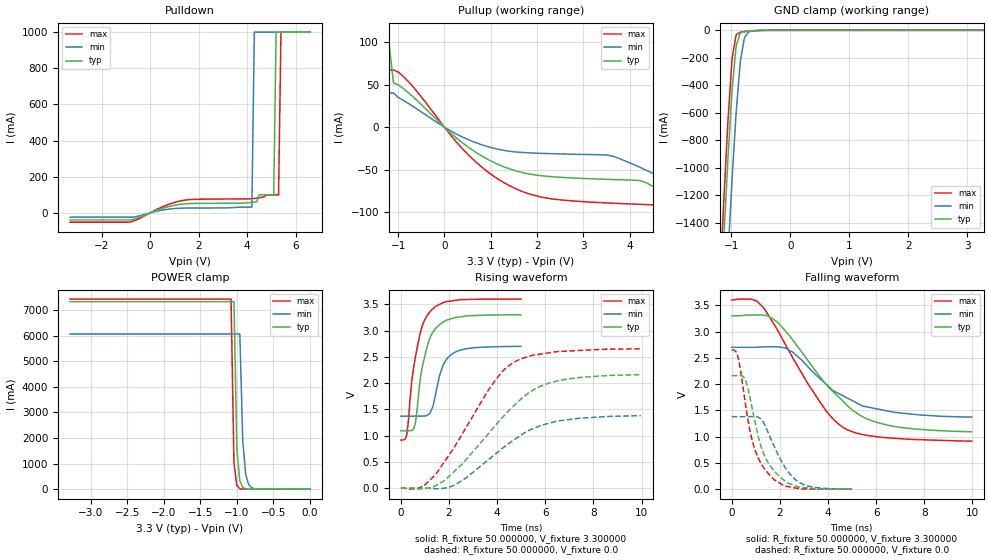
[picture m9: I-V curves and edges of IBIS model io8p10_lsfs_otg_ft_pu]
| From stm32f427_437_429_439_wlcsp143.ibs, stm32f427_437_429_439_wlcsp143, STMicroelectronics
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|   Model io8p10_lsfs_otg_ft_pu
[Model]  io8p10_lsfs_otg_ft_pu
Model_type I/O
Polarity   Non-Inverting
Enable   Active-Low
Vinl =   0.990000V
Vinh =   2.310000V
Vmeas =  1.650000V
Cref =   40.000000pF
Rref =   100.000000M
Vref =   0.0V
C_comp   8.196500pF   7.968500pF   8.492600pF
[Temperature Range]   25.000000   0.125000k   -40.000000
[Pullup Reference]   3.300000V   2.700000V   3.600000V
[Pulldown Reference]   0.0V   0.0V   0.0V
[POWER Clamp Reference]   3.300000V   2.700000V   3.600000V
[GND Clamp Reference]   0.0V   0.0V   0.0V
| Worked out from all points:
|   slope of the pulldown table from 0 to 0.495 V, typ, clamps not added: 20.1 ohm
|   slope of the pullup table from 0 to 0.495 V, typ, clamps not added: 21.8 ohm
|   GND clamp passes 1 mA (typ) near -0.52 V on its own axis
|   POWER clamp passes 1 mA (typ) near -0.80 V on its own axis
|   rising waveform, R_fixture 50.000000, V_fixture 3.300000: 20-80 % time 526ps typ, 499ps min, 529ps max; typ from 1.09 V to 3.3 V
|   rising waveform, R_fixture 50.000000, V_fixture 0.0: 20-80 % time 2.59ns typ, 2.41ns min, 2.19ns max; typ from 0.001 V to 2.16 V
|   falling waveform, R_fixture 50.000000, V_fixture 3.300000: 20-80 % time 2.44ns typ, 2.26ns min, 2.13ns max; typ from 3.3 V to 1.09 V
|   falling waveform, R_fixture 50.000000, V_fixture 0.0: 20-80 % time 849ps typ, 952ps min, 758ps max; typ from 2.16 V to 0.001 V
[Pulldown]
|Voltage   I(typ)   I(min)   I(max)
-3.3V     -38.65mA   -23.43mA   -51.3mA
-900mV    -38.65mA   -23.43mA   -51.3mA
1.4V      49.88mA    26.66mA    69.84mA
4.2V      58.43mA    32mA       78.86mA
4.3V      60.2mA     1A         80.13mA
4.4V      62mA       1A         81.72mA
4.5V      100mA      1A         83.79mA
5.1V      100mA      1A         100mA
5.2V      1A         1A         100mA
5.3V      1A         1A         100mA
5.4V      1A         1A         1A
6.6V      1A         1A         1A
[Pullup]
|Voltage   I(typ)   I(min)   I(max)
-3.3V     100mA      1A         67mA
-1.6V     100mA      1A         67mA
-1.5V     100mA      40mA       67mA
-1.2V     100mA      40mA       67mA
-1.1V     52mA       40mA       67mA
800mV     -33.66mA   -20.62mA   -46.63mA
2V        -56.45mA   -30.57mA   -80.98mA
3.5V      -61.24mA   -32.7mA    -88.93mA
4.2V      -62.55mA   -46.6mA    -90.52mA
4.9V      -82mA      -66mA      -102.3mA
5.5V      -103mA     -66mA      -126.2mA
6.6V      -103mA     -66mA      -139mA
[GND_clamp]
|Voltage   I(typ)   I(min)   I(max)
-3.3V     -9.479A    -9.465A    -9.974A
-1.2V     -2.125A    -2.854A    -1.857A
-1.13V    -1.511A    -2.236A    -1.236A
-1.06V    -933.3mA   -1.641A    -660.9mA
-990mV    -433.3mA   -1.082A    -206.9mA
-920mV    -110.3mA   -591mA     -31.45mA
-850mV    -19.78mA   -226.7mA   -13.65mA
-780mV    -8.311mA   -53.93mA   -9.506mA
-710mV    -5.285mA   -11.94mA   -6.262mA
-640mV    -3.232mA   -4.282mA   -3.577mA
3.28V     0A         0A         0A
[POWER_clamp]
|Voltage   I(typ)   I(min)   I(max)
-3.28V    7.329A     6.064A     7.43A
-1.08V    7.329A     6.064A     7.43A
-1.04V    7.329A     6.064A     1.015A
-1V       1.545A     6.064A     138.8mA
-960mV    325.8mA    6.064A     19.13mA
-920mV    68.77mA    1.89A      2.772mA
-880mV    14.59mA    589.1mA    520.3uA
-840mV    3.154mA    183.6mA    196.4uA
-800mV    734.4uA    57.27mA    136.6uA
-720mV    96.98uA    5.605mA    116.7uA
0V        0A         0A         0A
[Ramp]
| variable   typ   min   max
dV/dt_r  1.28451/2.59000n   0.82114/2.39692n   1.58763/2.18976n
dV/dt_f  1.29996/2.41613n   0.78216/2.23662n   1.59709/2.12461n
R_load = 50.000000
[Rising Waveform]
R_fixture= 50.000000
V_fixture= 3.300000
V_fixture_min= 2.700000
V_fixture_max= 3.600000
|time   V(typ)   V(min)   V(max)
0s        1.092V     1.372V     915.8mV
250.2ps   1.092V     1.372V     1.026V
460.5ps   1.1V       1.372V     2.071V
540.5ps   1.14V      1.372V     2.323V
610.6ps   1.262V     1.372V     2.511V
890.9ps   2.306V     1.372V     3.093V
1.251ns   2.902V     1.474V     3.38V
1.752ns   3.161V     2.343V     3.53V
2.142ns   3.234V     2.56V      3.567V
4.985ns   3.3V       2.7V       3.6V
[Rising Waveform]
R_fixture= 50.000000
V_fixture= 0.0
V_fixture_min= 0.0
V_fixture_max= 0.0
|time   V(typ)   V(min)   V(max)
0s        1.084mV    1.041mV    1.065mV
760.8ps   -15.37mV   1.053mV    5.82mV
1.441ns   47.59mV    -11.43mV   259.2mV
2.242ns   330mV      61.26mV    795.7mV
3.704ns   1.074V     566.8mV    1.913V
4.224ns   1.349V     760.4mV    2.224V
4.705ns   1.574V     921.8mV    2.4V
5.526ns   1.877V     1.14V      2.534V
6.466ns   2.038V     1.276V     2.599V
9.97ns    2.161V     1.38V      2.653V
[Falling Waveform]
R_fixture= 50.000000
V_fixture= 3.300000
V_fixture_min= 2.700000
V_fixture_max= 3.600000
|time   V(typ)   V(min)   V(max)
0s        3.3V       2.7V       3.6V
840.8ps   3.315V     2.7V       3.614V
1.341ns   3.308V     2.709V     3.444V
1.962ns   3.15V      2.706V     2.977V
2.543ns   2.833V     2.605V     2.495V
3.904ns   2.007V     2.004V     1.502V
4.625ns   1.673V     1.777V     1.177V
5.325ns   1.407V     1.609V     1.051V
6.346ns   1.232V     1.501V     982.7mV
9.97ns    1.092V     1.372V     915.8mV
[Falling Waveform]
R_fixture= 50.000000
V_fixture= 0.0
V_fixture_min= 0.0
V_fixture_max= 0.0
|time   V(typ)   V(min)   V(max)
0s        2.161V     1.38V      2.653V
250.2ps   2.163V     1.38V      2.536V
580.6ps   2.064V     1.38V      1.593V
750.8ps   1.764V     1.381V     1.122V
961ps     1.298V     1.38V      759.4mV
1.231ns   797.2mV    1.326V     481.7mV
1.522ns   497.7mV    1.07V      298.2mV
2.192ns   166.5mV    430.1mV    62.07mV
2.763ns   45.77mV    142.6mV    14.12mV
4.985ns   1.084mV    1.041mV    1.065mV
